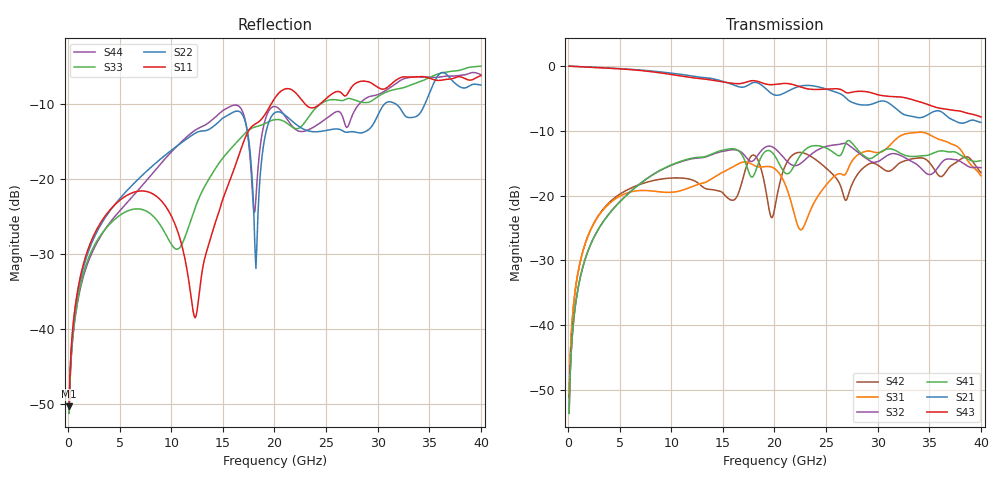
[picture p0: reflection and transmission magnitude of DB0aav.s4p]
! ADC12DJ2700AAV, ADC12DJ3200AAV, ADC08DJ3200AAV
! 144 pin AAV package
! Texas Instruments 4/21/2021
! Single-ended  S-parameters
! PORT#  PORT_NAME  NET_NAME
! PORT1:  DAxN.DIEBUMP DAxN
! PORT2:  DAxN.BGA  DAxN
! PORT3:  DAxP.DIEBUMP DAxP
! PORT4:  DAxP.BGA  DAxP
! Touchstone Ver. 1.0
! Number of ports is 4
# Hz	S	MA	R	50.000000
! SCATTERING PARAMETERS  :
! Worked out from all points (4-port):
!   400 points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, 100 MHz to 40 GHz, reference 50 ohm
!   strongest paths, dB at 100 MHz, 10.1 GHz, 20.1 GHz, 30.1 GHz, 40 GHz:
!     S43: 0.0, -1.3, -2.8, -4.5, -7.8
!     S21: 0.0, -1.1, -4.5, -5.5, -8.7
!     S41: -53.6, -15.2, -14.0, -13.5, -14.6
!     S32: -53.6, -15.3, -12.8, -14.7, -15.7
!     S31: -51.1, -19.5, -15.9, -13.4, -16.9
!     S42: -51.1, -17.3, -21.3, -15.4, -16.5
!   lowest |S11| = -50.3 dB at 100 MHz (marker M1), VSWR 1.01, Z = 50.2 + j0.259 ohm
!   |S11| at or under -10 dB: start of sweep to 19.67 GHz; 22.97 GHz to 24.4 GHz (1.425 GHz wide, 6.02 % of centre)
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1e8  0.003055 57.5  0.9981 -1.4  0.002778 85.4  0.002084 -95.0
     0.9981 -1.4  0.003038 57.5  0.002084 -95.0  0.002777 86.1
     0.002778 85.4  0.002084 -95.0  0.002751 55.6  0.9982 -1.3
     0.002084 -95.0  0.002777 86.1  0.9982 -1.3  0.002738 55.5
2e9  0.03501 43.2  0.9834 -25.5  0.05032 52.0  0.03859 -122.8
     0.9834 -25.5  0.03336 52.9  0.03868 -122.2  0.05045 67.1
     0.05032 52.0  0.03868 -122.2  0.02997 39.0  0.9824 -24.7
     0.03859 -122.8  0.05045 67.1  0.9824 -24.7  0.02858 46.0
8.4e9  0.07819 -70.3  0.9107 -105.0  0.1079 -85.9  0.1483 146.3
       0.9107 -105.0  0.1262 -9.6  0.1479 147.7  0.1314 15.1
       0.1079 -85.9  0.1479 147.7  0.05514 -93.2  0.898 -101.3
       0.1483 146.3  0.1314 15.1  0.898 -101.3  0.1139 -14.6
1.23e10  0.01187 142.7  0.8308 -152.6  0.1199 156.6  0.1965 85.4
         0.8308 -152.6  0.2019 -53.6  0.194 88.6  0.1293 -20.9
         0.1199 156.6  0.194 88.6  0.06395 74.9  0.8084 -145.2
         0.1965 85.4  0.1293 -20.9  0.8084 -145.2  0.2116 -60.3
1.82e10  0.2343 -25.3  0.7477 140.1  0.1685 31.1  0.1567 13.1
         0.7477 140.1  0.02536 39.2  0.1956 12.1  0.1997 37.8
         0.1685 31.1  0.1956 12.1  0.2235 -40.8  0.7676 151.8
         0.1567 13.1  0.1997 37.8  0.7676 151.8  0.07436 -118.7
2.19e10  0.3845 -95.4  0.6748 106.0  0.07316 -59.0  0.1692 -26.2
         0.6748 106.0  0.2373 136.0  0.1704 -41.8  0.2096 69.7
         0.07316 -59.0  0.1704 -41.8  0.2187 -83.1  0.7157 108.8
         0.1692 -26.2  0.2096 69.7  0.7157 108.8  0.2187 126.7
4e10  0.4901 37.2  0.3672 -104.0  0.1423 -12.4  0.1861 76.7
      0.3672 -104.0  0.4243 -81.9  0.1643 82.7  0.1503 -6.6
      0.1423 -12.4  0.1643 82.7  0.5666 75.0  0.4052 -95.9
      0.1861 76.7  0.1503 -6.6  0.4052 -95.9  0.497 -99.7
